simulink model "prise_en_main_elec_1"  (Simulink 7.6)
settings: Solver=ode15s  StartTime=0.0  StopTime=N  RelTol=1e-3
InitFcn:
  | close all
  | clc
  | N=20; % temps de simulation
  | R=1e3;    % 1 Kohm
  | C=1e-3;  % 1 mF
StopFcn:
  | load appli_circuit_RC.mat
  | plot(x(1,:),x(2,:),x(1,:),x(3,:))
  | title('Charge d''une capacité d''un circuit RC')
  | grid
  | axis([0 N -0.5 5.5])
  | xlabel('temps')
undefined symbols (not defined in the file or in its folder): sigbuilder_block
libraries: fl_lib x7, nesl_utility x4, elec_lib x1

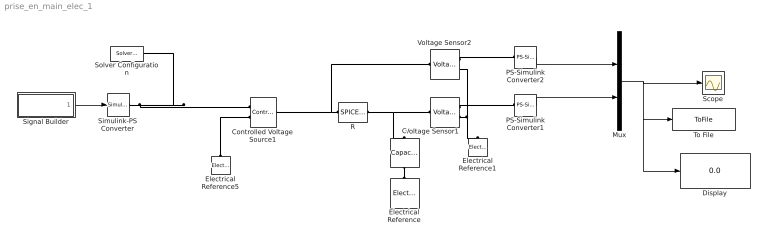
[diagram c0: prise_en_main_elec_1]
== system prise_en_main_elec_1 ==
  C : fl_lib/Electrical/Electrical Elements/Capacitor  DialogController=NetworkEngine.DynNeDlgSource  SystemSampleTime=-1  c=C F  v0=0 V  r=1e-06 Ohm  g=0 1/Ohm  i_Log=off  v_Log=off  vc_Log=off  LocalVarNames=|i|v|vc  LocalVarDescs=|i|v|Internal variable for voltage across capacitor term  LocalVarLogging=[0 0 0]
  Controlled Voltage Source1 : fl_lib/Electrical/Electrical Sources/Controlled Voltage Source  DialogController=NetworkEngine.DynNeDlgSource  SystemSampleTime=-1  i_Log=off  v_Log=off  LocalVarNames=|current|voltage|power  LocalVarDescs=|Current (A)|Voltage (V)|Power (W)  LocalVarLogging=[0 0 0]
  Display : Display
  Electrical Reference : fl_lib/Electrical/Electrical Elements/Electrical Reference  DialogController=NetworkEngine.DynNeDlgSource  SystemSampleTime=-1  i_Log=off  LocalVarNames=|i  LocalVarDescs=|i  LocalVarLogging=0
  Electrical Reference1 : fl_lib/Electrical/Electrical Elements/Electrical Reference  DialogController=NetworkEngine.DynNeDlgSource  SystemSampleTime=-1  i_Log=off  LocalVarNames=|i  LocalVarDescs=|i  LocalVarLogging=[]
  Electrical Reference5 : fl_lib/Electrical/Electrical Elements/Electrical Reference  DialogController=NetworkEngine.DynNeDlgSource  SystemSampleTime=-1  i_Log=off  LocalVarNames=|i  LocalVarDescs=|i  LocalVarLogging=[]
  Mux : Mux  Inputs=2
  PS-Simulink Converter1 : nesl_utility/PS-Simulink Converter  DialogController=NetworkEngine.DynNeUtilDlgSource  SystemSampleTime=-1  PhysicalDomain=network_engine_domain  LeftPortType=input  RightPortType=output  SubClassName=ps_output  Unit=1  AffineConversion=off
  PS-Simulink Converter2 : nesl_utility/PS-Simulink Converter  DialogController=NetworkEngine.DynNeUtilDlgSource  SystemSampleTime=-1  PhysicalDomain=network_engine_domain  LeftPortType=input  RightPortType=output  SubClassName=ps_output  Unit=1  AffineConversion=off
  R : elec_lib/Additional Components/SPICE-Compatible Components/Passive Devices/SPICE Resistor  DialogController=NetworkEngine.DynNeDlgSource  SystemSampleTime=-1  SCALE=1  R_param=1  R=R Ohm  RSH=0 Ohm  LENGTH=1e-06 m  WIDTH=1e-06 m  NARROW=0 m  T_param=1  TC1=0 1/K  TC2=0 1/K^2  TOFFSET=0 K  TFIXED=300.15 K  TMEAS=300.15 K  LocalVarLogging=[]
  Scope : Scope
  Signal Builder : Subsystem  Tag=STV Subsys  LoadFcn=sigbuilder_block('load');  StartFcn=sigbuilder_block('start');  StopFcn=sigbuilder_block('stop');  ClipboardFcn=sigbuilder_block('clipboard');
  Simulink-PS Converter : nesl_utility/Simulink-PS Converter  DialogController=NetworkEngine.DynNeUtilDlgSource  SystemSampleTime=-1  PhysicalDomain=network_engine_domain  LeftPortType=input  RightPortType=output  SubClassName=ps_input  Unit=1  AffineConversion=off  InputFilterTimeConstant=.001  UdotUserProvided=0
  Solver Configuration : nesl_utility/Solver Configuration  DialogController=NetworkEngine.DynNeUtilDlgSource  SystemSampleTime=-1  PhysicalDomain=network_engine_domain  LeftPortType=input  RightPortType=generic  SubClassName=solver  Accelerate=off  Profile=off  ResidualTolerance=1e-9  MaxNonlinIter=12  MaxModeIter=2  DoFixedCost=off  UseLocalSampling=off  DoDC=off  LinearAlgebra=Sparse  LocalSolverSampleTime=.001  LocalSolverChoice=NE_BACKWARD_EULER_ADVANCER  UseLocalSolver=off
  To File : ToFile  Filename=appli_circuit_RC  MatrixName=x
  Voltage Sensor1 : fl_lib/Electrical/Electrical Sensors/Voltage Sensor  DialogController=NetworkEngine.DynNeDlgSource  SystemSampleTime=-1  i1_Log=off  v1_Log=off  LocalVarNames=|i1|v1  LocalVarDescs=|i1|v1  LocalVarLogging=[]
  Voltage Sensor2 : fl_lib/Electrical/Electrical Sensors/Voltage Sensor  DialogController=NetworkEngine.DynNeDlgSource  SystemSampleTime=-1  i1_Log=off  v1_Log=off  LocalVarNames=|i1|v1  LocalVarDescs=|i1|v1  LocalVarLogging=[]
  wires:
  PS-Simulink Converter2/1 -> Mux/1
  Signal Builder/1(Signal 1) -> Simulink-PS Converter/1
  PS-Simulink Converter1/1 -> Mux/2
  Mux/1 -> Scope/1, To File/1, Display/1
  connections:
  R/RConn1 -- C/LConn1 -- Voltage Sensor1/LConn1
  C/RConn1 -- Electrical Reference/LConn1
  Voltage Sensor2/RConn1 -- PS-Simulink Converter2/LConn1
  Electrical Reference5/LConn1 -- Controlled Voltage Source1/RConn2
  Voltage Sensor2/LConn1 -- R/LConn1 -- Controlled Voltage Source1/LConn1
  Voltage Sensor1/RConn1 -- PS-Simulink Converter1/LConn1
  Voltage Sensor1/RConn2 -- Electrical Reference1/LConn1 -- Voltage Sensor2/RConn2
  Simulink-PS Converter/RConn1 -- Controlled Voltage Source1/RConn1 -- Solver Configuration/RConn1

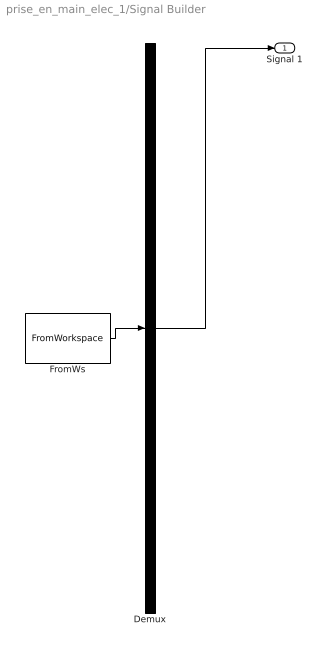
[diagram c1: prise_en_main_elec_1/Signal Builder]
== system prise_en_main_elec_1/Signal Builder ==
  Demux : Demux  Tag=STV Demux  Outputs=1
  FromWs : FromWorkspace  Tag=STV FromWs  VariableName=tuvar  SampleTime=0  SigBuilderData=DataTag0  VnvData=DataTag1
  Signal 1 : Outport  Tag=STV Outport
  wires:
  Demux/1 -> Signal 1/1
  FromWs/1 -> Demux/1
